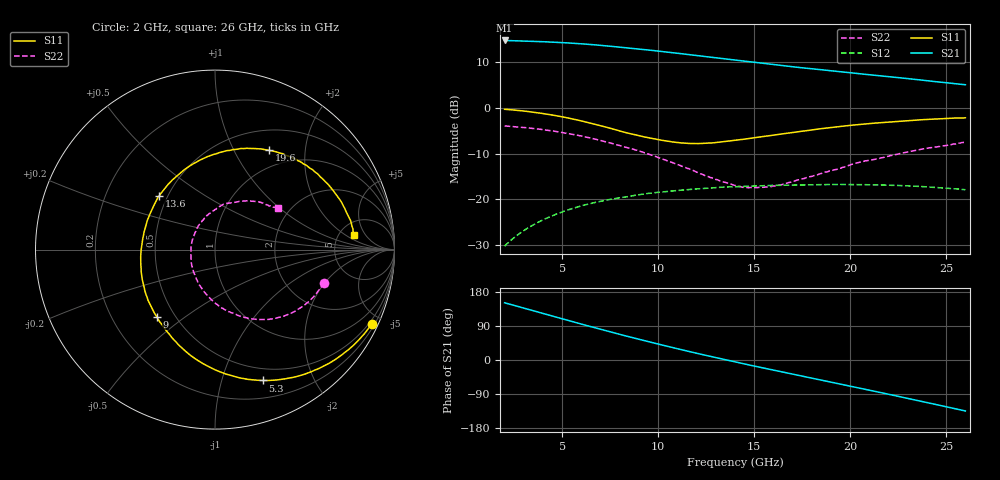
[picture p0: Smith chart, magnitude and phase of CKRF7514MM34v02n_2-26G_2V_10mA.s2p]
! CHUO DENSHI KOGYO Co.,Ltd.
! 22. July 2016
! CKRF7514MM34
! N-channel HJ-FET
! Vds = 2 V Id = 10 mA
# Hz S  MA  R 50
!	f	S11	S21	S12	S22
!	Hz	MAG	ANG	MAG	ANG	MAG	ANG	MAG	ANG
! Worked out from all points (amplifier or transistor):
!   241 points, 2 GHz to 26 GHz, reference 50 ohm
!   highest |S21| = 14.8 dB at 2 GHz (marker M1)
!   |S21| within 3 dB of that: start of sweep to 11.4 GHz
!   unconditionally stable (mu >= 1): 12.12 GHz to 19.47 GHz
!   at 6 GHz: K = 0.65, MSG = 17.8 dB, |S12| = -21.5 dB
!   at 14 GHz: K = 1.03, MAG = 12.8 dB, |S12| = -17.3 dB
!   at 26 GHz: K = 0.85, MSG = 11.5 dB, |S12| = -17.9 dB
!   lowest NFmin = 0.32 dB at 10 GHz
!   S11 on the Smith chart (normalised r, x): 2 GHz: 0.36, -4.43; 5.3 GHz: 0.37, -1.36; 9 GHz: 0.40, -0.39; 13.6 GHz: 0.45, +0.33; 19.6 GHz: 0.76, +1.39; 26 GHz: 6.85, +2.85
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2e9  0.9657 -25.3  5.476 151.0  0.0306 73.4  0.6339 -16.8
2.9e9  0.929 -37.0  5.406 138.4  0.04384 66.4  0.6124 -24.4
3.7e9  0.8847 -47.7  5.339 127.1  0.05527 60.0  0.5884 -31.4
4.5e9  0.8338 -58.7  5.25 115.8  0.06613 53.7  0.5588 -38.4
5.3e9  0.7757 -70.0  5.144 104.5  0.07645 47.3  0.5247 -45.7
6e9  0.7201 -80.4  5.033 94.8  0.08445 42.0  0.4922 -52.2
6.7e9  0.6629 -91.2  4.901 85.1  0.09201 36.5  0.456 -58.5
7.4e9  0.6064 -102.8  4.76 75.6  0.09873 31.3  0.418 -65.2
8.1e9  0.5514 -114.8  4.601 66.2  0.1044 26.2  0.38 -71.9
9e9  0.4951 -131.0  4.407 54.7  0.112 20.5  0.3374 -81.2
1e10  0.4489 -151.3  4.19 42.0  0.1192 13.5  0.2857 -92.6
1.08e10  0.4222 -168.1  4.01 32.2  0.1237 8.3  0.2486 -102.3
1.17e10  0.4073 172.9  3.812 21.3  0.1283 2.5  0.2104 -115.5
1.26e10  0.4109 154.5  3.619 10.9  0.132 -3.0  0.1772 -130.8
1.36e10  0.4316 136.0  3.415 -0.5  0.1364 -9.2  0.1503 -151.7
1.4e10  0.4411 129.0  3.336 -5.0  0.1372 -11.8  0.1415 -160.3
1.6e10  0.5028 100.4  2.983 -26.8  0.1414 -23.5  0.1394 150.9
1.8e10  0.5734 77.3  2.683 -47.9  0.1443 -35.3  0.178 111.4
1.96e10  0.6303 61.5  2.477 -64.9  0.1449 -45.4  0.2232 90.1
2.2e10  0.7003 39.9  2.197 -90.4  0.1424 -61.5  0.2958 64.2
2.39e10  0.7455 22.9  1.996 -111.3  0.1366 -75.6  0.3592 47.9
2.6e10  0.7792 6.0  1.792 -134.6  0.1271 -92.2  0.42 33.4
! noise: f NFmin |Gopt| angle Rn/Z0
1e+10  0.32  0.442  101.8  0.06
1.05e+10  0.34  0.418  109.7  0.06
1.1e+10  0.36  0.387  119.5  0.05
1.15e+10  0.38  0.359  129.9  0.05
1.2e+10  0.41  0.334  141.6  0.04
1.25e+10  0.42  0.313  155.2  0.04
1.3e+10  0.44  0.3  168.6  0.04
1.35e+10  0.46  0.295  -177.5  0.04
1.4e+10  0.49  0.303  -162.9  0.04
1.5e+10  0.53  0.324  -140.6  0.05
